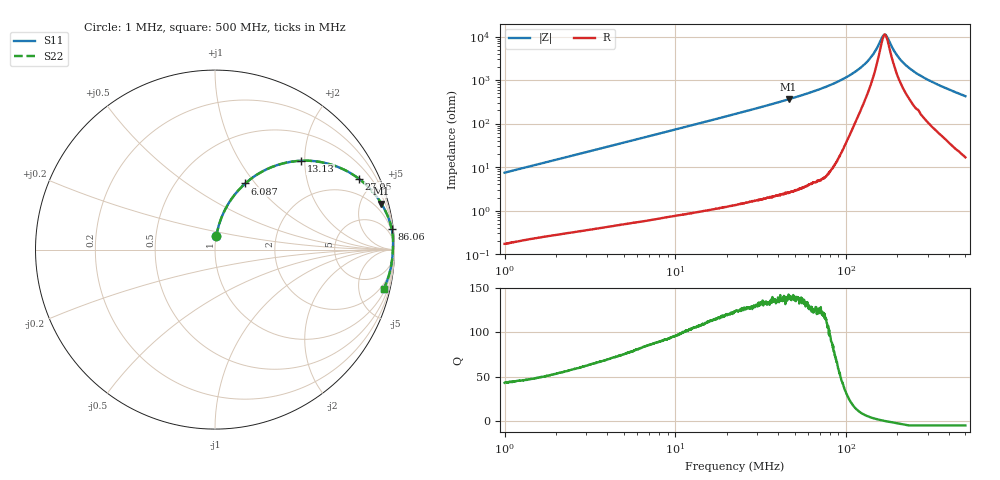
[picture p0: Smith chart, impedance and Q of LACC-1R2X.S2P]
!s-Parameter Generated by FASTRON Sdn. Bhd.
!FASTRON P/N : LACC-1R2X
!Keysight Technologies,E4991B,MY54100416,A.01.15
!Date: Wed Mar 18 08:56:52 2026
!Version  : Rev00 Wed Mar 18 08:56:52 2026
!Data & Calibration Information:
!PortZ  Port1:50+j0  Port2:50+j0
!When reading, reference impedance value at option line is always used.
!Remarks : This data is being provided solely for informational purposes.
!Freq	S11	S21	S12	S22
# Hz S dB R 50
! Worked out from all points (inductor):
!   1601 points, 1 MHz to 500 MHz, reference 50 ohm
!   read as one part in series: L = 1.18 uH near 1.032 MHz
!   highest Q = 140 at 46.05 MHz (marker M1), where L = 1.25 uH
!   self-resonance near 168.9 MHz
!   S11 on the Smith chart (normalised r, x): 1 MHz: 1.00, +0.15; 6.087 MHz: 1.01, +0.89; 13.13 MHz: 1.02, +1.92; 27.05 MHz: 1.03, +4.03; 86.06 MHz: 1, +17; 500 MHz: 1.34, -8.51
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1000000  -22.59 84.4  -0.04 -4.3  -0.04 -4.3  -22.59 84.4
2820919  -13.87 77.4  -0.21 -11.7  -0.21 -11.7  -13.87 77.4
6086788  -7.85 65.4  -0.83 -23.9  -0.83 -23.9  -7.85 65.4
7957584  -6.01 59.3  -1.31 -30.1  -1.31 -30.1  -6.01 59.3
1.313366e7  -3.22 45.8  -2.89 -43.6  -2.89 -43.6  -3.22 45.8
2.236068e7  -1.38 31.0  -5.75 -58.5  -5.75 -58.5  -1.38 31.0
2.704836e7  -0.98 26.3  -7.07 -63.3  -7.07 -63.3  -0.98 26.3
4.605113e7  -0.34 15.5  -11.48 -74.1  -11.48 -74.1  -0.34 15.5
6.307767e7  -0.16 10.6  -14.69 -78.9  -14.69 -78.9  -0.16 10.6
8.606451e7  -0.07 6.7  -18.71 -82.6  -18.71 -82.6  -0.07 6.7
1.086514e8  -0.06 4.1  -22.96 -82.9  -22.96 -82.9  -0.06 4.1
1.294029e8  -0.06 2.4  -27.59 -79.1  -27.59 -79.1  -0.06 2.4
1.453951e8  -0.07 1.3  -32.31 -70.2  -32.31 -70.2  -0.07 1.3
1.659216e8  -0.08 0.2  -40.68 -17.1  -40.68 -17.1  -0.08 0.2
1.711582e8  -0.08 -0.1  -40.73 12.2  -40.73 12.2  -0.08 -0.1
1.77937e8  -0.08 -0.4  -38.34 39.8  -38.34 39.8  -0.08 -0.4
1.908225e8  -0.09 -1.1  -33.60 61.6  -33.60 61.6  -0.09 -1.1
2.046412e8  -0.09 -1.7  -30.15 69.9  -30.15 69.9  -0.09 -1.7
2.220328e8  -0.10 -2.4  -27.19 74.2  -27.19 74.2  -0.10 -2.4
2.475421e8  -0.11 -3.5  -24.21 77.0  -24.21 77.0  -0.11 -3.5
3.312556e8  -0.15 -6.7  -18.66 78.3  -18.66 78.3  -0.15 -6.7
5e8  -0.31 -13.1  -12.90 74.7  -12.90 74.7  -0.31 -13.1
